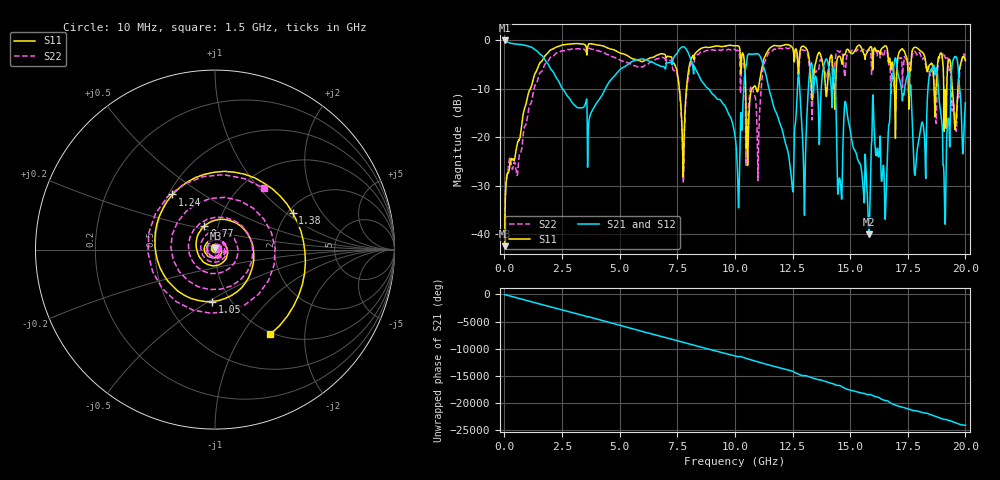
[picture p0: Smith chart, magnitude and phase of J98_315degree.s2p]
!Keysight Technologies,N5222A,MY51421036,A.10.65.16
!Date: Friday, March 31, 2023 15:18:47
!Correction: S11(Full 2 Port(1,2))
!S21(Full 2 Port(1,2))
!S12(Full 2 Port(1,2))
!S22(Full 2 Port(1,2))
!S2P File: Measurements: S11, S21, S12, S22:
# Hz S  dB  R 50
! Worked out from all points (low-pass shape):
!   2000 points, 10 MHz to 20 GHz, reference 50 ohm
!   highest |S21| = 0.00 dB at 10 MHz (marker M1); lowest = -40.0 dB at 15.81 GHz (marker M2)
!   |S21| within 3 dB of the highest: start of sweep to 1.603 GHz; 7.428 GHz to 8.013 GHz (585.6 MHz wide, 7.59 % of centre)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
!   lowest |S11| = -42.4 dB at 10 MHz (marker M3), VSWR 1.02, Z = 50.2 + j0.723 ohm
!   |S11| at or under -10 dB: start of sweep to 1.12 GHz; 7.593 GHz to 7.898 GHz (304.8 MHz wide, 3.94 % of centre); 10.47 GHz to 10.74 GHz (271.1 MHz wide, 2.56 % of centre)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
!   |S22| runs from -38.0 to -1.5 dB; largest |S21 - S12| = 0.012
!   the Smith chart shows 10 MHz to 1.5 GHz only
!   S11 on the Smith chart (normalised r, x): 10 MHz: 1.00, +0.01; 770 MHz: 0.86, +0.23; 1.05 GHz: 0.82, -0.52; 1.24 GHz: 0.52, +0.38; 1.38 GHz: 2.12, +1.13; 1.5 GHz: 0.97, -1.34
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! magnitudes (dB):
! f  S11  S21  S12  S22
! 10 MHz  -42.4  0.0  0.0  -37.4
! 770 MHz  -16.8  -0.9  -0.9  -21.7
! 1.05 GHz  -10.8  -1.2  -1.2  -14.3
! 1.24 GHz  -8.2  -1.6  -1.6  -11.2
! 1.38 GHz  -6.4  -2.0  -2.0  -8.9
! 1.5 GHz  -5.0  -2.6  -2.6  -7.2
! 3.35 GHz  -0.7  -13.9  -13.9  -1.8
! 6.68 GHz  -2.9  -5.1  -5.1  -3.8
! 7.75 GHz  -27.2  -1.3  -1.3  -26.6
! 8.17 GHz  -3.2  -5.2  -5.2  -4.4
! 10.01 GHz  -1.1  -19.8  -19.8  -1.9
! 11.01 GHz  -10.1  -2.8  -2.8  -26.7
! 12.46 GHz  -1.3  -28.8  -28.7  -1.6
! 13.34 GHz  -11.5  -4.9  -4.9  -16.2
! 15.81 GHz  -1.8  -40.0  -39.5  -1.9
! 16.67 GHz  -4.5  -17.8  -17.8  -5.0
! 16.96 GHz  -20.1  -3.6  -3.6  -14.4
! 17.83 GHz  -1.4  -27.1  -27.1  -2.3
! 18.56 GHz  -4.9  -5.8  -5.9  -5.7
! 19.1 GHz  -11.9  -34.5  -34.4  -3.2
! 19.5 GHz  -14.3  -3.6  -3.6  -13.5
! 20 GHz  -4.2  -12.8  -12.7  -3.9
